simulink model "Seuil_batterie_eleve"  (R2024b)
settings: Solver=VariableStepAuto  StartTime=0.0  StopTime=400000  RelTol=1e-3
libraries: ee_lib x5, nesl_utility x4, fl_lib x3, simulink x2, batteryecm_lib x1, simulink_extras x1

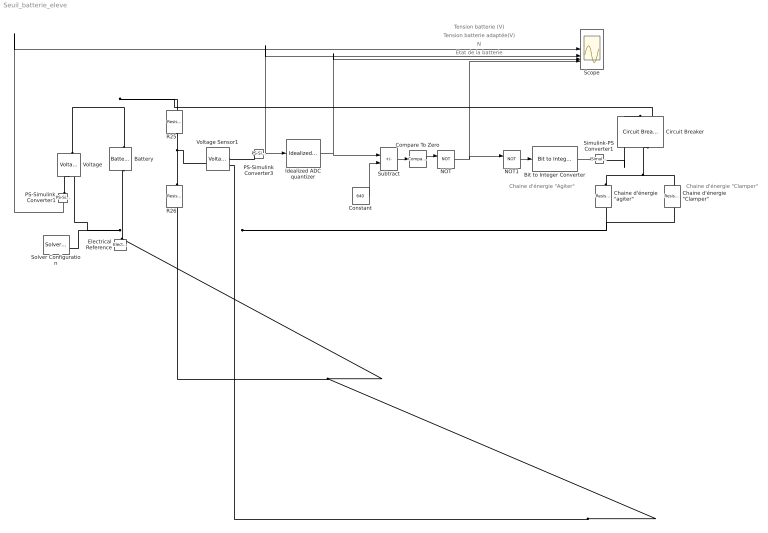
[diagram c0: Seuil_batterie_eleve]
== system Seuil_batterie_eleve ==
  note: Chaine d'énergie "Agiter"
  note: N
  note: Tension batterie (V)
  note: Etat de la batterie
  note: Chaine d'énergie "Clamper"
  note: Tension batterie adaptée(V)
  Battery : batteryecm_lib/Battery  Vnom=12 V  prm_dir=simscape.enum.battery.prm_dir.disabled  R1_dis=2 Ohm  R1_ch=2 Ohm  R1=0.2 Ohm  prm_AH=2  AH=3.8 Ah  V1=10.8 V  AH1=0.8 hr*A  prm_R2=1  R2=2000 Ohm  Tmeas=298.15 K  charge_measurement_port=simscape.enum.battery.enable.no  prm_dyn=1  Rp1=0.005 Ohm  tau1=30 s  Rp2=0.005 Ohm  tau2=30 s  Rp3=0.005 Ohm  tau3=30 s  Rp4=0.005 Ohm  tau4=30 s  Rp5=0.005 Ohm  tau5=30 s  prm_fade=1  N_fade=100  AH_fade=45 hr*A  R1_fade=2.02 Ohm  R1_ch_fade=2.02 Ohm  V1_fade=10.35 V  prm_age=simscape.enum.battery.prm_age.disabled  prm_age_OCV=simscape.enum.battery.prm_age_OCV.OCV  OCV_age=0.9  SOC_age=60  Tmeas_age=298.15 K  delta_time_age_vec=[0] d  temperature_age_vec=[273] K  OCV_scaling_age=2.2134e6  OCV_offset_age=1.632e6  temp_exp_age=0.515833569 V  t_exp_age=0.75  Vnom_T2=12 V  R1_T2=2.2 Ohm  R1_T2_dis=2.2 Ohm  R1_T2_ch=2.2 Ohm  V1_T2=11.4 V  R2_T2=2200 Ohm  Rp1_T2=0.005 Ohm  tau1_T2=30 s  Rp2_T2=0.005 Ohm  tau2_T2=30 s  Rp3_T2=0.005 Ohm  tau3_T2=30 s  Rp4_T2=0.005 Ohm  tau4_T2=30 s  Rp5_T2=0.005 Ohm  tau5_T2=30 s  Tmeas2=273.15 K  thermal_port=simscape.enum.thermaleffects.omit  thermal_mass=30000 J/K  i_specify=off  i_priority=None  i=0 A  i_nominal_specify=off  i_nominal_value=1  i_nominal_unit=A  v_specify=off  v_priority=None  v=14 V  v_nominal_specify=off  v_nominal_value=1  v_nominal_unit=V  charge_specify=on  charge_priority=High  charge=3.8 hr*A  charge_nominal_specify=off  charge_nominal_value=1  charge_nominal_unit=hr*A  num_cycles_specify=off  num_cycles_priority=High  num_cycles=0  num_cycles_nominal_specify=off  num_cycles_nominal_value=1  num_cycles_nominal_unit=1  temperature_specify=off  temperature_priority=High  temperature=298.15 K  temperature_nominal_specify=off  temperature_nominal_value=1  temperature_nominal_unit=K
  Bit to Integer Converter : simulink/Logic and Bit Operations/Bit to Integer Converter  nbits=1  bitOrder=MSB first  signedOutputValues=Unsigned  outDtype=double  outDtypeSigned=Inherit via internal rule
  "Chaine d'énergie \"Clamper\"" : ee_lib/Passive/Resistor  R=500 Ohm  enable_R_tol=1  R_tol=0.1  tol_distribution=1  nSigma=4  enable_operating_limits=0  operating_limit_action=2  power_rating=1 W  max_working_voltage=100 V  noise_mode=0  Tdevice=25 degC  sample_time=1e-3 s  repeatability=1  user_seed=0  auto_seed=233087700  fault_action=simscape.enum.assert.action.none  t_fault=1 s  power_derating_T1=70 degC  power_derating_T2=155 degC  operating_temperature_range_vec=[-50, 150] degC  alpha=3.93e-3 1/K  Tmeas=25 degC  thermal_mass=100 J/K  temperature_specify=off  temperature_priority=High  temperature=298.15 K  temperature_nominal_specify=off  temperature_nominal_value=1  temperature_nominal_unit=K
  "Chaine d'énergie \"agiter\"" : ee_lib/Passive/Resistor  R=500 Ohm  enable_R_tol=1  R_tol=0.1  tol_distribution=1  nSigma=4  enable_operating_limits=0  operating_limit_action=2  power_rating=1 W  max_working_voltage=100 V  noise_mode=0  Tdevice=25 degC  sample_time=1e-3 s  repeatability=1  user_seed=0  auto_seed=569266544  fault_action=simscape.enum.assert.action.none  t_fault=1 s  power_derating_T1=70 degC  power_derating_T2=155 degC  operating_temperature_range_vec=[-50, 150] degC  alpha=3.93e-3 1/K  Tmeas=25 degC  thermal_mass=100 J/K  temperature_specify=off  temperature_priority=High  temperature=298.15 K  temperature_nominal_specify=off  temperature_nominal_value=1  temperature_nominal_unit=K
  Circuit Breaker : ee_lib/Switches & Breakers/Circuit Breaker  R_closed=0.001 Ohm  G_open=1e-6 1/Ohm  threshold=0.5 V  breaker_behavior=ee.enum.switches.breakerBehavior.zeroCrossingDisable
  Compare To Zero : simulink/Logic and Bit Operations/Compare To Zero  relop=<=  OutDataTypeStr=boolean
  Constant : Constant  Value=640
  Electrical Reference : fl_lib/Electrical/Electrical Elements/Electrical Reference
  Idealized ADC quantizer : simulink_extras/Additional Discrete/Idealized ADC quantizer  NumberOfConverterBits=12  Vmin=0  Vmax=2.5  OutputDataType=uint32  OutputNegativeValues=off
  NOT : Logic  Operator=NOT  IconShape=distinctive  AllPortsSameDT=off  OutDataTypeStr=boolean
  NOT1 : Logic  Operator=NOT  IconShape=distinctive  AllPortsSameDT=off  OutDataTypeStr=boolean
  PS-Simulink Converter1 : nesl_utility/PS-Simulink Converter  PhysicalDomain=network_engine_domain  SubClassName=ps_output  LeftPortType=input  RightPortType=output  PseudoPeriodic=off  Frequencies=[]  VectorFormat=1-D array  Unit=inherit  AffineConversion=off
  PS-Simulink Converter3 : nesl_utility/PS-Simulink Converter  PhysicalDomain=network_engine_domain  SubClassName=ps_output  LeftPortType=input  RightPortType=output  PseudoPeriodic=off  Frequencies=[]  VectorFormat=1-D array  Unit=inherit  AffineConversion=off
  R25 : ee_lib/Passive/Resistor  R=10 kOhm  enable_R_tol=1  R_tol=0.1  tol_distribution=1  nSigma=4  enable_operating_limits=0  operating_limit_action=2  power_rating=1 W  max_working_voltage=100 V  noise_mode=0  Tdevice=25 degC  sample_time=1e-3 s  repeatability=1  user_seed=0  auto_seed=2474800446  fault_action=simscape.enum.assert.action.none  t_fault=1 s  power_derating_T1=70 degC  power_derating_T2=155 degC  operating_temperature_range_vec=[-50, 150] degC  alpha=3.93e-3 1/K  Tmeas=25 degC  thermal_mass=100 J/K  temperature_specify=off  temperature_priority=High  temperature=298.15 K  temperature_nominal_specify=off  temperature_nominal_value=1  temperature_nominal_unit=K
  R26 : ee_lib/Passive/Resistor  R=10 kOhm  enable_R_tol=1  R_tol=0.1  tol_distribution=1  nSigma=4  enable_operating_limits=0  operating_limit_action=2  power_rating=1 W  max_working_voltage=100 V  noise_mode=0  Tdevice=25 degC  sample_time=1e-3 s  repeatability=1  user_seed=0  auto_seed=2243586  fault_action=simscape.enum.assert.action.none  t_fault=1 s  power_derating_T1=70 degC  power_derating_T2=155 degC  operating_temperature_range_vec=[-50, 150] degC  alpha=3.93e-3 1/K  Tmeas=25 degC  thermal_mass=100 J/K  temperature_specify=off  temperature_priority=High  temperature=298.15 K  temperature_nominal_specify=off  temperature_nominal_value=1  temperature_nominal_unit=K
  Scope : Scope  NumInputPorts=4
  Simulink-PS Converter1 : nesl_utility/Simulink-PS Converter  PhysicalDomain=network_engine_domain  SubClassName=ps_input  LeftPortType=input  RightPortType=output  PseudoPeriodic=off  Frequencies=[]  NoiseDistribution=none  NoiseParameters=[]  Unit=1  AffineConversion=off  FilteringAndDerivatives=provide  SimscapeFilterOrder=1  InputFilterTimeConstant=0.001  UdotUserProvided=0
  Solver Configuration : nesl_utility/Solver Configuration  PhysicalDomain=network_engine_domain  SubClassName=solver  LeftPortType=input  RightPortType=generic  Tones=[]  Harmonics=[]  SimulateNoise=off  Profile=off  UseLocalSampling=off  EnableSwitchedLinearOptims=on  FrequencyDomain=off  UseCCode=off  RelTol=0.001  AbsTol=1e-06  MinStep=1e-09  ToWorkspace=off  RevertToSquareIcSolve=off  NumHomotopyIterations=100  PhasorMode=off  PhasorModeNumHarmonics=1  ConsistencySolver=NEWTON_FTOL  IndexReductionMethod=DerivativeReplacement  DoDC=off  ResidualTolerance=1e-09  ConsistencyTolSource=GLOBAL  ConsistencyAbsTol=0.001  ConsistencyRelTol=0.001  ConsistencyTolFactor=0.001  UseLocalSolver=off  LocalSolverChoice=NE_BACKWARD_EULER_ADVANCER  ResolveIndetEquations=on  FunctionEvalNumThread=1  LocalSolverSampleTime=0.001  DoFixedCost=off  MaxNonlinIter=3  MaxModeIter=2  ComputeImpulses=off  ImpulseIterations=2  LinearAlgebra=auto  LinearAlgebraNumThread=0  EquationFormulation=NE_TIME_EF  DelaysMemoryBudget=1024  AutomaticFiltering=on  FilteringTimeConstant=0.001  PartitionStorageMethod=AS_NEEDED  PartitionMemoryBudget=1024  PartitionMethod=ROBUST  MultibodyUseLocalSolver=off  MultibodyLocalSolverChoice=ODE1  MultibodyLocalSolverSampleTime=0.001
  Subtract : Sum  Inputs=+-
  Voltage : fl_lib/Electrical/Electrical Sensors/Voltage Sensor
  Voltage Sensor1 : fl_lib/Electrical/Electrical Sensors/Voltage Sensor
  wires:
  PS-Simulink Converter3/1 -> Scope/2, Idealized ADC quantizer/1
  Constant/1 -> Subtract/2
  Idealized ADC quantizer/1 -> Scope/3, Subtract/1
  Subtract/1 -> Compare To Zero/1
  Compare To Zero/1 -> NOT/1
  NOT/1 -> Scope/4, NOT1/1
  PS-Simulink Converter1/1 -> Scope/1
  NOT1/1 -> Bit to Integer Converter/1
  Bit to Integer Converter/1 -> Simulink-PS Converter1/1
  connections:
  Voltage/LConn1 -- R25/LConn1 -- Circuit Breaker/LConn2 -- Battery/LConn1
  R25/RConn1 -- Voltage Sensor1/LConn1 -- R26/LConn1
  PS-Simulink Converter3/LConn1 -- Voltage Sensor1/RConn1
  Electrical Reference/LConn1 -- Solver Configuration/RConn1 -- Voltage/RConn2 -- "Chaine d'énergie \"agiter\""/RConn1 -- "Chaine d'énergie \"Clamper\""/RConn1 -- Voltage Sensor1/RConn2 -- R26/RConn1 -- Battery/RConn1
  PS-Simulink Converter1/LConn1 -- Voltage/RConn1
  Circuit Breaker/LConn1 -- Simulink-PS Converter1/RConn1
  "Chaine d'énergie \"agiter\""/LConn1 -- "Chaine d'énergie \"Clamper\""/LConn1 -- Circuit Breaker/RConn1
